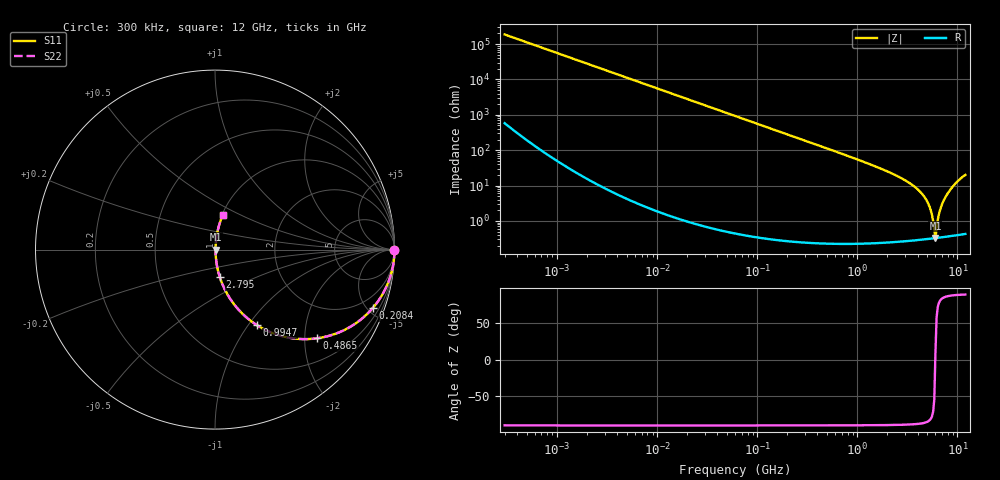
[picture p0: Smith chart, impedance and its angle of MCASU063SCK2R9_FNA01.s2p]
! MCASU063SCK2R9_FNA01  S-PARAMETER MODEL  ( General Type )
! Model Generated by TAIYO YUDEN Corporation (http://www.ty-top.com)
! Version 1.0
! TAIYO YUDEN Control No. 130801
! Copyright(c) 2013 TAIYO YUDEN CO.,LTD. All Rights Reserved.
! Product Description (link to TY-COMPAS)
! https://ds.yuden.co.jp/TYCOMPAS/or/detail?pn=MCASU063SCK2R9CFNA01&u=M
! Products Name : Multilayer Ceramic Capacitors
! Characteristics :
!  Capacitance : 2.9 pF , Rated Voltage : 50V , TCC : CK / C0K
!  Case Size : 0.6 x 0.3 / 0.024 x 0.012 [mm/inch] , Thickness : 0.3 / 0.012 [mm/inch]
!  (Conditions: Temperature = 25 degC , DC Bias Current/Voltage = 0A / 0V)
! External Node Assignments :
!  1  o---| |---o  2
! GND o---------o GND
! Frequency Range : 0.3MHz  -  12000MHz  [ 401 STEP ]
# MHz S RI R 50
! Freq[MHz].  S11 Real  S11 Imag  S21 Real  S21 Imag  S12 Real  S12 Imag  S22 Real  S22 Imag
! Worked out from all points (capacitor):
!   401 points, 300 kHz to 12 GHz, reference 50 ohm
!   read as one part in series: C = 2.83 pF near 316.3 kHz
!   lowest |Z| = 330 mohm at 6.026 GHz (marker M1)
!   series resonance near 6.01 GHz, so ESL is about 250 pH
!   S11 on the Smith chart (normalised r, x): 300 kHz: open; 208.4 MHz: 1.01, -5.39; 486.5 MHz: 1.00, -2.30; 994.7 MHz: 1.00, -1.10; 2.795 GHz: 1.01, -0.32; 12 GHz: 1.01, +0.40
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0.3  1 -0.000533  1.93e-06 0.000533  1.93e-06 0.000533  1 -0.000533
1.769972  1 -0.00315  1.17e-05 0.00315  1.17e-05 0.00315  1 -0.00315
10.44266  0.9996 -0.0186  0.00035 0.0186  0.00035 0.0186  0.9996 -0.0186
60  0.9887 -0.1054  0.0113 0.1054  0.0113 0.1054  0.9887 -0.1054
208.3979  0.8789 -0.3258  0.1211 0.3258  0.1211 0.3258  0.8789 -0.3258
353.9943  0.7148 -0.4508  0.2852 0.4508  0.2852 0.4508  0.7148 -0.4508
486.4723  0.5689 -0.4942  0.4311 0.4942  0.4311 0.4942  0.5689 -0.4942
994.7115  0.2333 -0.4209  0.7667 0.4209  0.7667 0.4209  0.2333 -0.4209
2088.533  0.0552 -0.2233  0.9448 0.2233  0.9448 0.2233  0.0552 -0.2233
2795.104  0.0267 -0.1532  0.9733 0.1532  0.9733 0.1532  0.0267 -0.1532
3740.715  0.0112 -0.0909  0.9888 0.0909  0.9888 0.0909  0.0112 -0.0909
4623.766  0.00542 -0.0493  0.9946 0.0493  0.9946 0.0493  0.00542 -0.0493
5278.635  0.0037 -0.0242  0.9963 0.0242  0.9963 0.0242  0.0037 -0.0242
5715.274  0.00328 -0.0094  0.9967 0.0094  0.9967 0.0094  0.00328 -0.0094
5868.704  0.00324 -0.00449  0.9968 0.00449  0.9968 0.00449  0.00324 -0.00449
6026.253  0.00325 0.000528  0.9967 -0.000528  0.9967 -0.000528  0.00325 0.000528
6188.031  0.00331 0.00511  0.9967 -0.00511  0.9967 -0.00511  0.00331 0.00511
6354.153  0.00341 0.00993  0.9966 -0.00993  0.9966 -0.00993  0.00341 0.00993
6879.757  0.00404 0.0252  0.996 -0.0252  0.996 -0.0252  0.00404 0.0252
7648.807  0.0059 0.0484  0.9941 -0.0484  0.9941 -0.0484  0.0059 0.0484
9454.42  0.0159 0.1087  0.9841 -0.1087  0.9841 -0.1087  0.0159 0.1087
12000  0.0421 0.1905  0.9579 -0.1905  0.9579 -0.1905  0.0421 0.1905
